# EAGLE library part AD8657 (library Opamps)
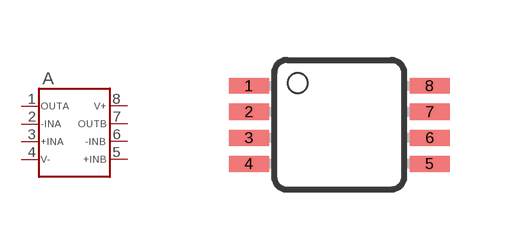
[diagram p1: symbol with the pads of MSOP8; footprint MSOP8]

Designator prefix A

## AD8657  [MSOP8]
1  OUTA  out
2  -INA  in
3  +INA  in
4  V-  in
5  +INB  in
6  -INB  in
7  OUTB  out
8  V+  in

## Footprint MSOP8 (pad centres in mm)
smd 1 x 0.4: 1 -2.263,0.976; 2 -2.263,0.326; 3 -2.263,-0.324; 4 -2.263,-0.974; 5 2.262,-0.974; 6 2.262,-0.324; 7 2.262,0.326; 8 2.262,0.976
